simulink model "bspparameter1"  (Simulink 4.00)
settings: Solver=ode45  SolverMode=SingleTasking  StartTime=0.0  StopTime=500.0  FixedStep=0.01  RelTol=1e-3
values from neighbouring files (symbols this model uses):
  Konst = 1.15    [bspparameter_ini.m]
  verst = 10    [bspparameter_ini.m]
libraries: simulink3 x1

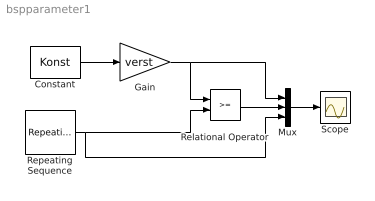
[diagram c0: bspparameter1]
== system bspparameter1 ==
  Constant : Constant  Value=Konst
  Gain : Gain  Gain=verst  Multiplication=Element-wise(K.*u)  SaturateOnIntegerOverflow=on
  Mux : Mux  Inputs=3
  Relational Operator : RelationalOperator  Operator=>=
  Repeating Sequence : simulink3/Sources/Repeating Sequence  rep_seq_t=zeit  rep_seq_y=wiederhol
  Scope : Scope
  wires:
  Relational Operator/1 -> Mux/2
  Repeating Sequence/1 -> Relational Operator/2, Mux/3
  Constant/1 -> Gain/1
  Gain/1 -> Relational Operator/1, Mux/1
  Mux/1 -> Scope/1
